(* Logix 5000 AddOnInstructionDefinition export SPEL_Above; software revision 30.01 *)

ADD_ON_INSTRUCTION SPEL_ExecCmd   (* revision 1.0 *)
// Executes a command in the robot controller.  Normally this is called by higher level AOIs.
VAR_INPUT
   Start : BOOL; {required}
   MaxTime : DINT := 3000; {required}
END_VAR
VAR_OUTPUT
   InCycle : BOOL; {access Read Only, visible}
   Done : BOOL; {access Read Only, visible}
   Error : BOOL; {access Read Only, visible}
END_VAR
VAR_IN_OUT
   ExtInputs : AB:ETHERNET_MODULE_INT_128Bytes:I:0; {required}
        .DATA[0].0   // ExtCmdGet
        .DATA[0].1   // ExtRespSet
        .DATA[0].2   // ExtCmdResult
        .DATA[0].3   // ExtError
   ExtOutputs : AB:ETHERNET_MODULE_INT_128Bytes:O:0; {required}
        .DATA[0].0   // ExtCmdSet
        .DATA[0].1   // ExtRespGet
        .DATA[0].2   // ExtCmdReset
END_VAR
VAR_INPUT
   Cmd : INT; {required}
   CmdParam1 : INT; {required}
   CmdParam2 : INT; {required}
   CmdParam3 : INT; {required}
   CmdParam4 : INT; {required}
   CmdParam5 : INT; {required}
   CmdParam6 : INT; {required}
   CmdParam7 : INT; {required}
END_VAR
VAR_OUTPUT
   CmdEcho : INT; {access Read Only, visible}
   Resp1 : INT; {access Read Only, visible}
   Resp2 : INT; {access Read Only, visible}
   Resp3 : INT; {access Read Only, visible}
   Resp4 : INT; {access Read Only, visible}
   Resp5 : INT; {access Read Only, visible}
   Resp6 : INT; {access Read Only, visible}
   Resp7 : INT; {access Read Only, visible}
   ErrCode1 : INT; {access Read Only, visible}
   ErrCode2 : INT; {access Read Only, visible}
END_VAR
VAR
   ExtReset : BOOL; {access None}
   ExtError : BOOL; {access None}
   ExtCmdSet : BOOL; {access None}   // Cmd Ready
   ExtCmdGet : BOOL; {access None}   // Cmd Received
   CmdXferDone : BOOL; {access None}
   ExtRespSet : BOOL; {access None}   // Resp Ready
   RespXferDone : BOOL; {access None}
   ExtCmdResult : BOOL; {access None}   // Normal or Error?
   TmrCmdDataRdy : TIMER := (PRE := 5); {access None}
   OneShotDoneOff : BOOL; {access None}
   OneShotStart : BOOL; {access None}
   StartInit : BOOL; {access None}
   OneShotStartError : BOOL; {access None}
   TmrCycle : TIMER := (PRE := 5000); {access None}
   OneshotTmrPreset : BOOL; {access None}
   TmrCmdSet : TIMER := (PRE := 20); {access None}
   OnShotCmdDataXfer : BOOL; {access None}
   OneShotRespDataXfer : BOOL; {access None}
   OneShotDataRdy : BOOL; {access None}
   OtherCmdInCycle : BOOL; {access None}
   s : BOOL; {access None}
   OneShotUnsetCmdIncycle : BOOL; {access None}
   OneShotSetCmdIncycle : BOOL; {access None}
   OneShotSetOtherCmdInCycleError : BOOL; {access None}
   OneShotSetBit : BOOL; {access None}
   MaxTimeError : BOOL; {access None}
END_VAR

ROUTINE Logic   (* ladder *)
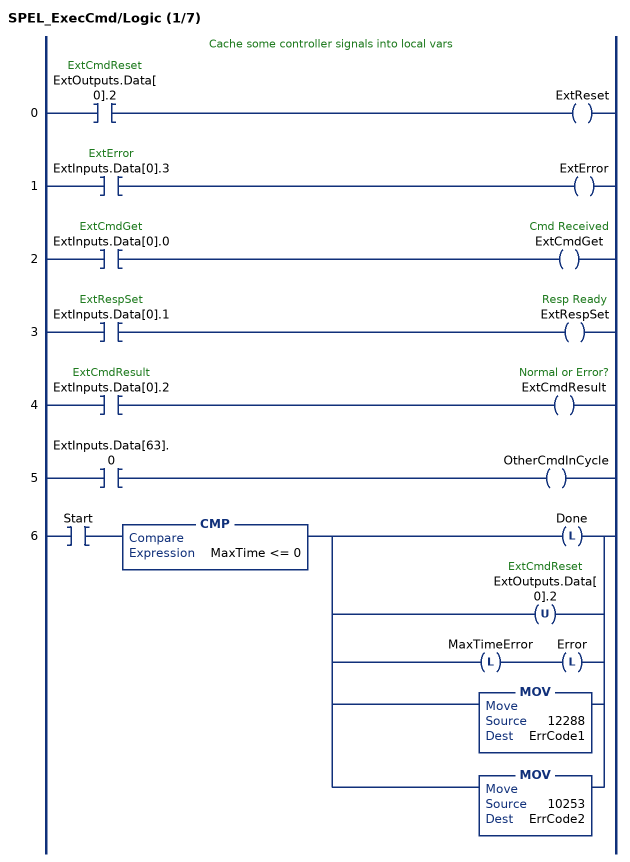
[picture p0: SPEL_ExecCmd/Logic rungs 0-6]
   // Cache some controller signals into local vars
   0: XIC(ExtOutputs.Data[0].2)OTE(ExtReset);
   1: XIC(ExtInputs.Data[0].3)OTE(ExtError);
   2: XIC(ExtInputs.Data[0].0)OTE(ExtCmdGet);
   3: XIC(ExtInputs.Data[0].1)OTE(ExtRespSet);
   4: XIC(ExtInputs.Data[0].2)OTE(ExtCmdResult);
   5: XIC(ExtInputs.Data[63].0)OTE(OtherCmdInCycle);
   6: XIC(Start)CMP(MaxTime <= 0)[OTL(Done) ,OTU(ExtOutputs.Data[0].2) ,OTL(MaxTimeError) OTL(Error) ,MOV(12288,ErrCode1) ,MOV(10253,ErrCode2) ];
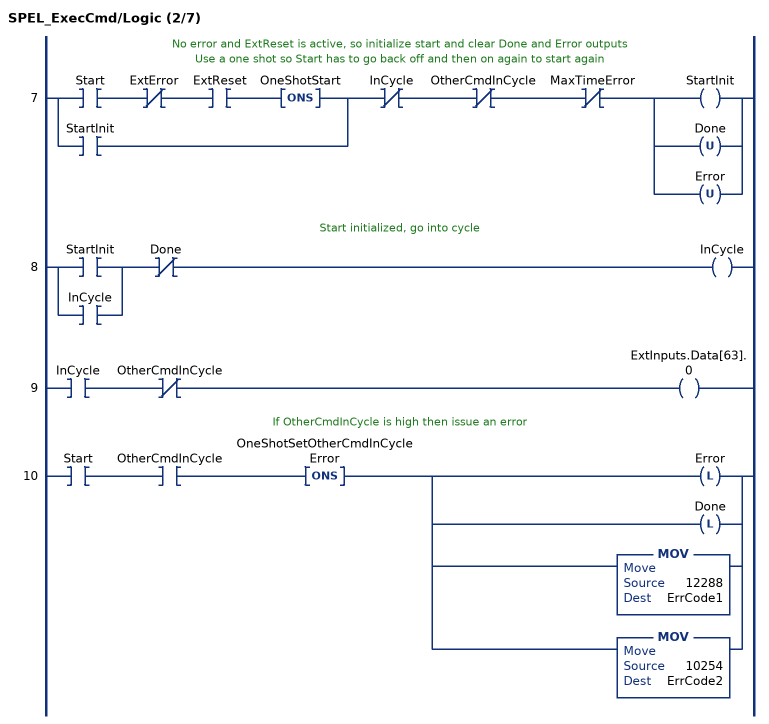
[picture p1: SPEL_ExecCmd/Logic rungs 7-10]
   // No error and ExtReset is active, so initialize start and clear Done and Error outputs
   // Use a one shot so Start has to go back off and then on again to start again
   7: [XIC(Start) XIO(ExtError) XIC(ExtReset) ONS(OneShotStart) ,XIC(StartInit) ]XIO(InCycle)XIO(OtherCmdInCycle)XIO(MaxTimeError)[OTE(StartInit) ,OTU(Done) ,OTU(Error) ];
   // Start initialized, go into cycle
   8: [XIC(StartInit) ,XIC(InCycle) ]XIO(Done)OTE(InCycle);
   9: XIC(InCycle)XIO(OtherCmdInCycle)OTE(ExtInputs.Data[63].0);
   // If OtherCmdInCycle is high then issue an error
   10: XIC(Start)XIC(OtherCmdInCycle)ONS(OneShotSetOtherCmdInCycleError)[OTL(Error) ,OTL(Done) ,MOV(12288,ErrCode1) ,MOV(10254,ErrCode2) ];
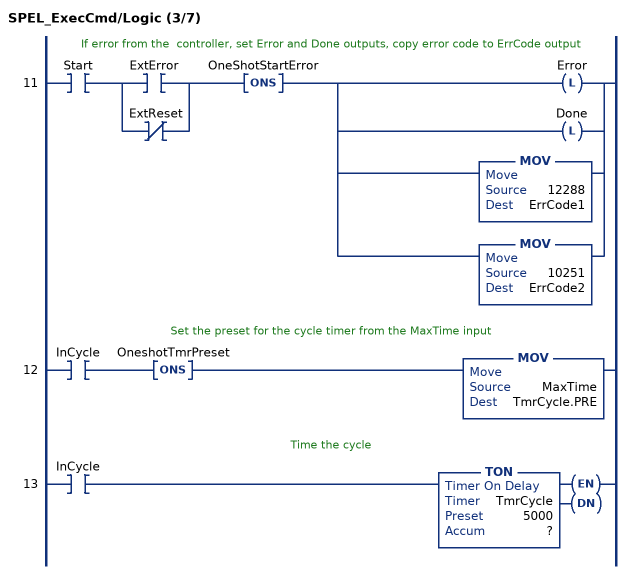
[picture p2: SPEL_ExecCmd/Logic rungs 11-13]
   // If error from the  controller, set Error and Done outputs, copy error code to ErrCode output
   11: XIC(Start)[XIC(ExtError) ,XIO(ExtReset) ]ONS(OneShotStartError)[OTL(Error) ,OTL(Done) ,MOV(12288,ErrCode1) ,MOV(10251,ErrCode2) ];
   // Set the preset for the cycle timer from the MaxTime input
   12: XIC(InCycle)ONS(OneshotTmrPreset)MOV(MaxTime,TmrCycle.PRE);
   // Time the cycle
   13: XIC(InCycle)TON(TmrCycle,?,?);
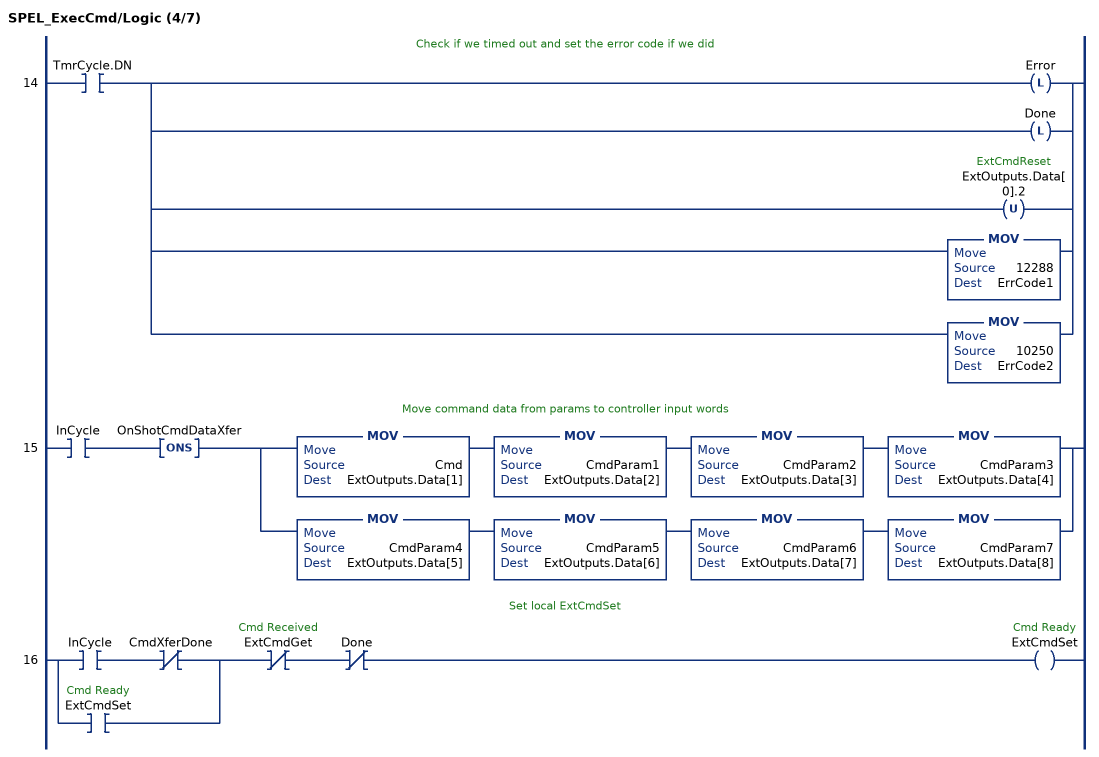
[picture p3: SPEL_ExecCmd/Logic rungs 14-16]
   // Check if we timed out and set the error code if we did
   14: XIC(TmrCycle.DN)[OTL(Error) ,OTL(Done) ,OTU(ExtOutputs.Data[0].2) ,MOV(12288,ErrCode1) ,MOV(10250,ErrCode2) ];
   // Move command data from params to controller input words
   15: XIC(InCycle)ONS(OnShotCmdDataXfer)[MOV(Cmd,ExtOutputs.Data[1]) MOV(CmdParam1,ExtOutputs.Data[2]) MOV(CmdParam2,ExtOutputs.Data[3]) MOV(CmdParam3,ExtOutputs.Data[4]) ,MOV(CmdParam4,ExtOutputs.Data[5]) MOV(CmdParam5,ExtOutputs.Data[6]) MOV(CmdParam6,ExtOutputs.Data[7]) MOV(CmdParam7,ExtOutputs.Data[8]) ];
   // Set local ExtCmdSet
   16: [XIC(InCycle) XIO(CmdXferDone) ,XIC(ExtCmdSet) ]XIO(ExtCmdGet)XIO(Done)OTE(ExtCmdSet);
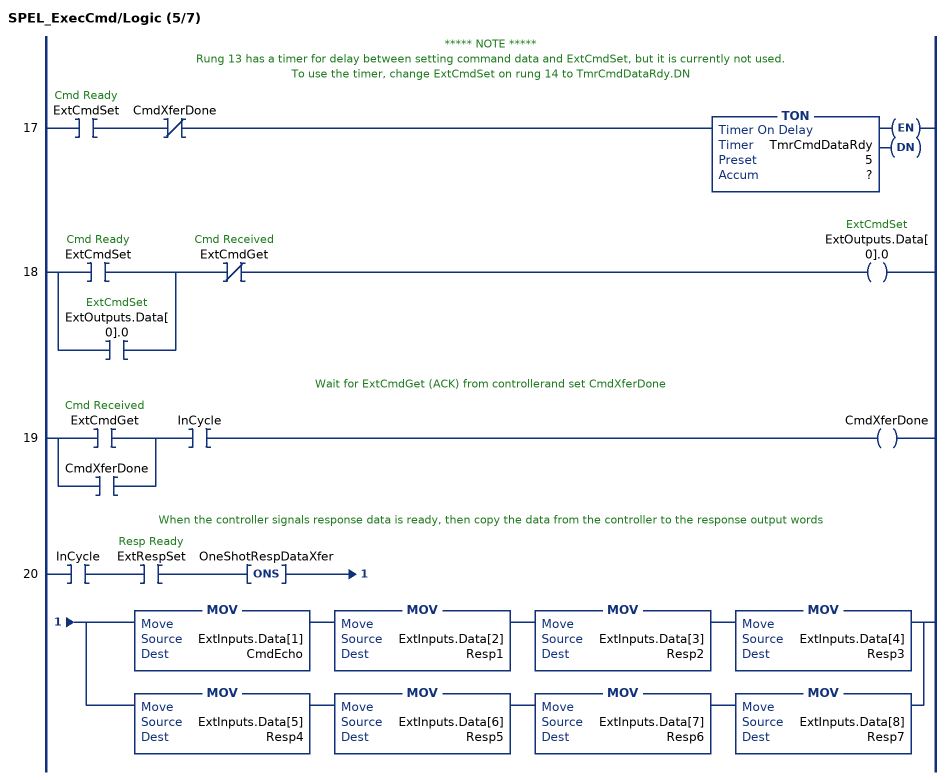
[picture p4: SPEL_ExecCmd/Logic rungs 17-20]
   // ***** NOTE *****
   // Rung 13 has a timer for delay between setting command data and ExtCmdSet, but it is currently not used.
   // To use the timer, change ExtCmdSet on rung 14 to TmrCmdDataRdy.DN
   17: XIC(ExtCmdSet)XIO(CmdXferDone)TON(TmrCmdDataRdy,?,?);
   18: [XIC(ExtCmdSet) ,XIC(ExtOutputs.Data[0].0) ]XIO(ExtCmdGet)OTE(ExtOutputs.Data[0].0);
   // Wait for ExtCmdGet (ACK) from controllerand set CmdXferDone
   19: [XIC(ExtCmdGet) ,XIC(CmdXferDone) ]XIC(InCycle)OTE(CmdXferDone);
   // When the controller signals response data is ready, then copy the data from the controller to the response output words
   20: XIC(InCycle)XIC(ExtRespSet)ONS(OneShotRespDataXfer)[MOV(ExtInputs.Data[1],CmdEcho) MOV(ExtInputs.Data[2],Resp1) MOV(ExtInputs.Data[3],Resp2) MOV(ExtInputs.Data[4],Resp3) ,MOV(ExtInputs.Data[5],Resp4) MOV(ExtInputs.Data[6],Resp5) MOV(ExtInputs.Data[7],Resp6) MOV(ExtInputs.Data[8],Resp7) ];
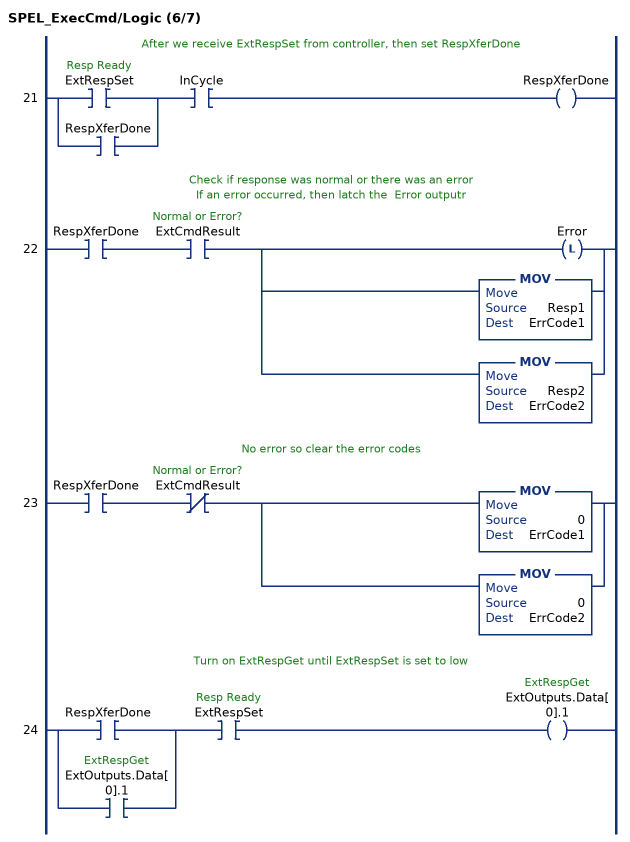
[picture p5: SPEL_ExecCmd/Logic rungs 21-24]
   // After we receive ExtRespSet from controller, then set RespXferDone
   21: [XIC(ExtRespSet) ,XIC(RespXferDone) ]XIC(InCycle)OTE(RespXferDone);
   // Check if response was normal or there was an error
   // If an error occurred, then latch the  Error outputr
   22: XIC(RespXferDone)XIC(ExtCmdResult)[OTL(Error) ,MOV(Resp1,ErrCode1) ,MOV(Resp2,ErrCode2) ];
   // No error so clear the error codes
   23: XIC(RespXferDone)XIO(ExtCmdResult)[MOV(0,ErrCode1) ,MOV(0,ErrCode2) ];
   // Turn on ExtRespGet until ExtRespSet is set to low
   24: [XIC(RespXferDone) ,XIC(ExtOutputs.Data[0].1) ]XIC(ExtRespSet)OTE(ExtOutputs.Data[0].1);
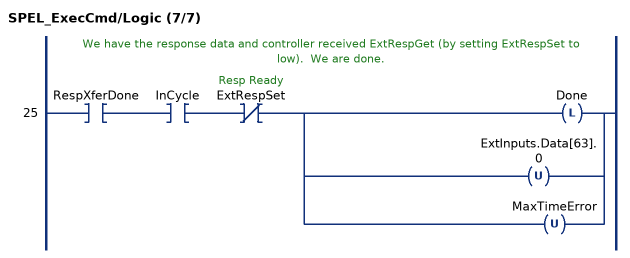
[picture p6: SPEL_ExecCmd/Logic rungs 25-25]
   // We have the response data and controller received ExtRespGet (by setting ExtRespSet to low).  We are done.
   25: XIC(RespXferDone)XIC(InCycle)XIO(ExtRespSet)[OTL(Done) ,OTU(ExtInputs.Data[63].0) ,OTU(MaxTimeError) ];
END_ROUTINE
END_ADD_ON_INSTRUCTION

ADD_ON_INSTRUCTION SPEL_Above   (* revision 1.0, vendor SEIKO EPSON CORP. *)
// Sets the elbow orientation of the specified point to ABOVE.
VAR_INPUT
   Start : BOOL; {required}
END_VAR
VAR_OUTPUT
   InCycle : BOOL; {access Read Only, visible}
   Done : BOOL; {access Read Only, visible}
   Error : BOOL; {access Read Only, visible}
END_VAR
VAR_INPUT
   Point : INT; {required}
END_VAR
VAR_IN_OUT
   ExtInputs : AB:ETHERNET_MODULE_INT_128Bytes:I:0; {required}
   ExtOutputs : AB:ETHERNET_MODULE_INT_128Bytes:O:0; {required}
END_VAR
VAR_OUTPUT
   ErrCode1 : INT; {access Read Only, visible}
   ErrCode2 : INT; {access Read Only, visible}
END_VAR
VAR
   ExecAbove : SPEL_ExecCmd := (MaxTime := 3000); {access None}
   StartCoil : BOOL; {access None}
   ExecTimeout : DINT; {access None}
   OneShotStart : BOOL; {access None}
END_VAR

ROUTINE Logic   (* ladder *)
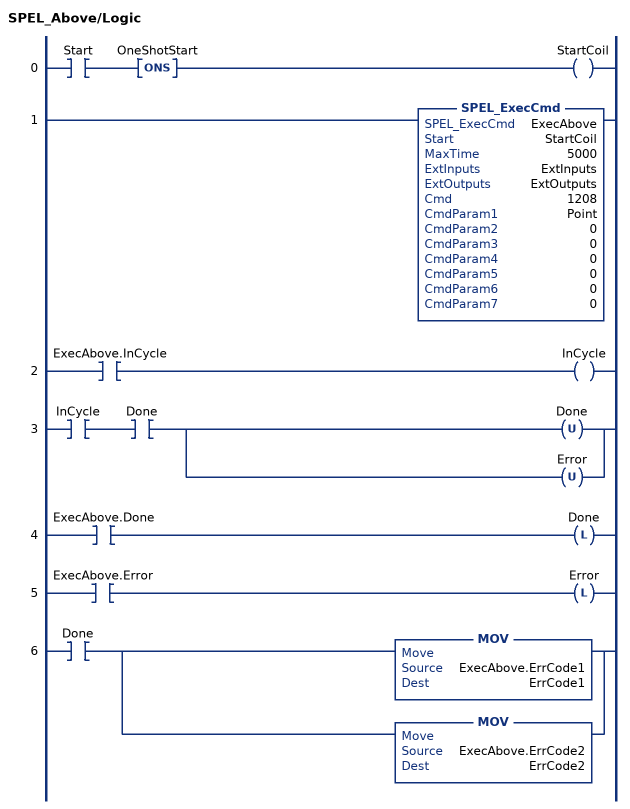
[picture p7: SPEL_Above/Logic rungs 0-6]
   0: XIC(Start)ONS(OneShotStart)OTE(StartCoil);
   1: SPEL_ExecCmd(ExecAbove,StartCoil,5000,ExtInputs,ExtOutputs,1208,Point,0,0,0,0,0,0);
   2: XIC(ExecAbove.InCycle)OTE(InCycle);
   3: XIC(InCycle)XIC(Done)[OTU(Done) ,OTU(Error) ];
   4: XIC(ExecAbove.Done)OTL(Done);
   5: XIC(ExecAbove.Error)OTL(Error);
   6: XIC(Done)[MOV(ExecAbove.ErrCode1,ErrCode1) ,MOV(ExecAbove.ErrCode2,ErrCode2) ];
END_ROUTINE
END_ADD_ON_INSTRUCTION

ADD_ON_INSTRUCTION SPEL_Accel   (* revision 1.0, vendor SEIKO EPSON CORP. *)
// Sets the point to point acceleration and deceleration for the current robot.  Accel and Decel inputs are a percentage.
VAR_INPUT
   Start : BOOL; {required}
END_VAR
VAR_OUTPUT
   InCycle : BOOL; {access Read Only, visible}
   Done : BOOL; {access Read Only, visible}
   Error : BOOL; {access Read Only, visible}
END_VAR
VAR_INPUT
   Accel : INT; {required}
   Decel : INT; {required}
END_VAR
VAR_IN_OUT
   ExtInputs : AB:ETHERNET_MODULE_INT_128Bytes:I:0; {required}
   ExtOutputs : AB:ETHERNET_MODULE_INT_128Bytes:O:0; {required}
END_VAR
VAR_OUTPUT
   ErrCode1 : INT; {access Read Only, visible}
   ErrCode2 : INT; {access Read Only, visible}
END_VAR
VAR
   ExecAccel : SPEL_ExecCmd := (MaxTime := 3000); {access None}   // Execute Accel Cmd
        .INCYCLE   // ExecInCycle
        .DONE   // ExecDone
        .ERROR   // ExecError
   OneShotStart : BOOL; {access None}
   StartCoil : BOOL; {access None}
   ExecTimeout : DINT; {access None}
END_VAR

ROUTINE Logic   (* ladder *)
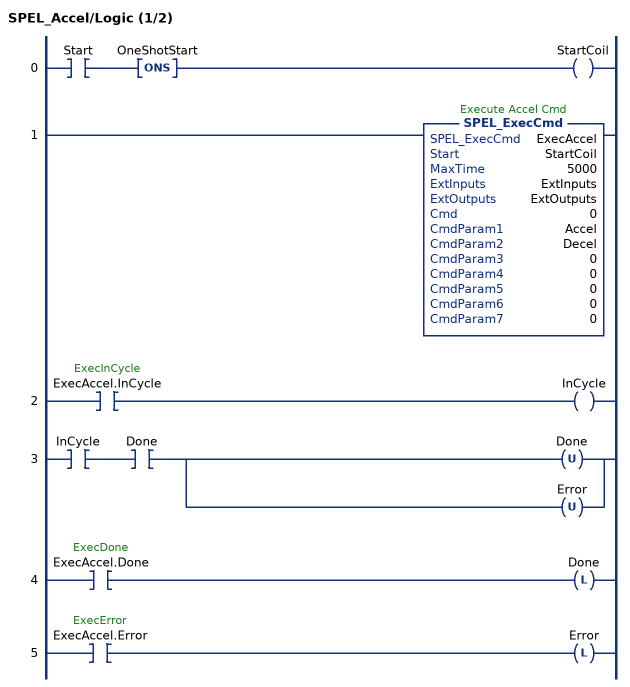
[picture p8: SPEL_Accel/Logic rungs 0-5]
   0: XIC(Start)ONS(OneShotStart)OTE(StartCoil);
   1: SPEL_ExecCmd(ExecAccel,StartCoil,5000,ExtInputs,ExtOutputs,0,Accel,Decel,0,0,0,0,0);
   2: XIC(ExecAccel.InCycle)OTE(InCycle);
   3: XIC(InCycle)XIC(Done)[OTU(Done) ,OTU(Error) ];
   4: XIC(ExecAccel.Done)OTL(Done);
   5: XIC(ExecAccel.Error)OTL(Error);
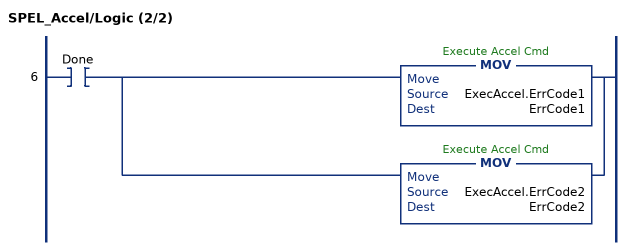
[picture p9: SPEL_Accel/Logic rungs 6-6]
   6: XIC(Done)[MOV(ExecAccel.ErrCode1,ErrCode1) ,MOV(ExecAccel.ErrCode2,ErrCode2) ];
END_ROUTINE
END_ADD_ON_INSTRUCTION

ADD_ON_INSTRUCTION SPEL_AccelS   (* revision 1.0, vendor SEIKO EPSON CORP. *)
// Sets linear motion acceleration and deceleration.
VAR_INPUT
   Start : BOOL; {required}
END_VAR
VAR_OUTPUT
   InCycle : BOOL; {access Read Only, visible}
   Done : BOOL; {access Read Only, visible}
   Error : BOOL; {access Read Only, visible}
END_VAR
VAR_INPUT
   Accel : REAL; {required}
   Decel : REAL; {required}
END_VAR
VAR_IN_OUT
   ExtInputs : AB:ETHERNET_MODULE_INT_128Bytes:I:0; {required}
   ExtOutputs : AB:ETHERNET_MODULE_INT_128Bytes:O:0; {required}
END_VAR
VAR_OUTPUT
   ErrCode1 : INT; {access Read Only, visible}
   ErrCode2 : INT; {access Read Only, visible}
END_VAR
VAR
   ExecAccelS : SPEL_ExecCmd := (MaxTime := 3000); {access None}
   Decel_INTS : INT[2]; {access None}
   Decelx1000 : DINT; {access None}
   OneShotStart : BOOL; {access None}
   StartInit : BOOL; {access None}
   Accel_INTS : INT[2]; {access None}
   Accelx1000 : DINT; {access None}
   ExecTimeout : DINT; {access None}
END_VAR

ROUTINE Logic   (* ladder *)
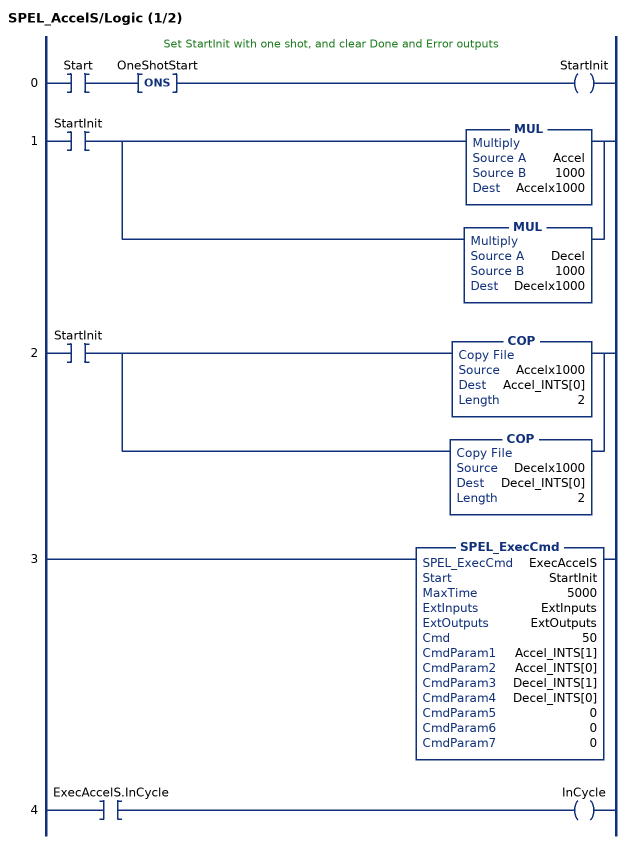
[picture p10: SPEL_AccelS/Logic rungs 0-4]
   // Set StartInit with one shot, and clear Done and Error outputs
   0: XIC(Start)ONS(OneShotStart)OTE(StartInit);
   1: XIC(StartInit)[MUL(Accel,1000,Accelx1000) ,MUL(Decel,1000,Decelx1000) ];
   2: XIC(StartInit)[COP(Accelx1000,Accel_INTS[0],2) ,COP(Decelx1000,Decel_INTS[0],2) ];
   3: SPEL_ExecCmd(ExecAccelS,StartInit,5000,ExtInputs,ExtOutputs,50,Accel_INTS[1],Accel_INTS[0],Decel_INTS[1],Decel_INTS[0],0,0,0);
   4: XIC(ExecAccelS.InCycle)OTE(InCycle);
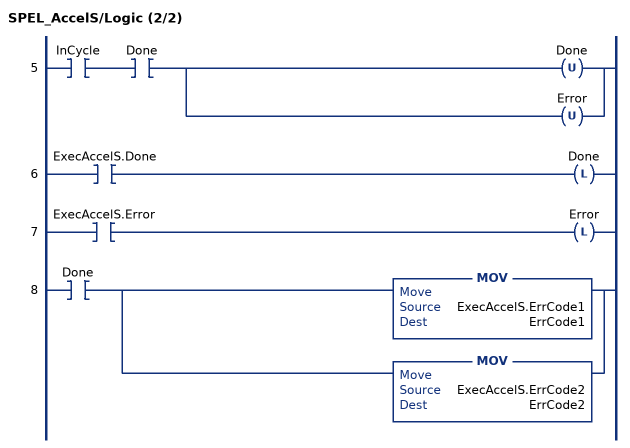
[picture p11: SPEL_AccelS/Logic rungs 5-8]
   5: XIC(InCycle)XIC(Done)[OTU(Done) ,OTU(Error) ];
   6: XIC(ExecAccelS.Done)OTL(Done);
   7: XIC(ExecAccelS.Error)OTL(Error);
   8: XIC(Done)[MOV(ExecAccelS.ErrCode1,ErrCode1) ,MOV(ExecAccelS.ErrCode2,ErrCode2) ];
END_ROUTINE
END_ADD_ON_INSTRUCTION

ADD_ON_INSTRUCTION SPEL_Arc   (* revision 1.0, vendor SEIKO EPSON CORP. *)
// Moves the arm from the current position to the specified position in circular interpolation motion on XY plane face.
VAR_INPUT
   Start : BOOL; {required}
   MaxTime : DINT := 10000; {access None, visible}
END_VAR
VAR_OUTPUT
   InCycle : BOOL; {access Read Only, visible}
   Done : BOOL; {access Read Only, visible}
   Error : BOOL; {access Read Only, visible}
END_VAR
VAR_INPUT
   MidPoint : INT; {required}
   EndPoint : INT; {required}
END_VAR
VAR_IN_OUT
   ExtInputs : AB:ETHERNET_MODULE_INT_128Bytes:I:0; {required}
   ExtOutputs : AB:ETHERNET_MODULE_INT_128Bytes:O:0; {required}
END_VAR
VAR_OUTPUT
   ErrCode1 : INT; {access Read Only, visible}
   ErrCode2 : INT; {access Read Only, visible}
END_VAR
VAR
   ExecArc : SPEL_ExecCmd := (MaxTime := 3000); {access None}
   StartCoil : BOOL; {access None}
   ExecTimeout : DINT; {access None}
   OneShotStart : BOOL; {access None}
END_VAR

ROUTINE Logic   (* ladder *)
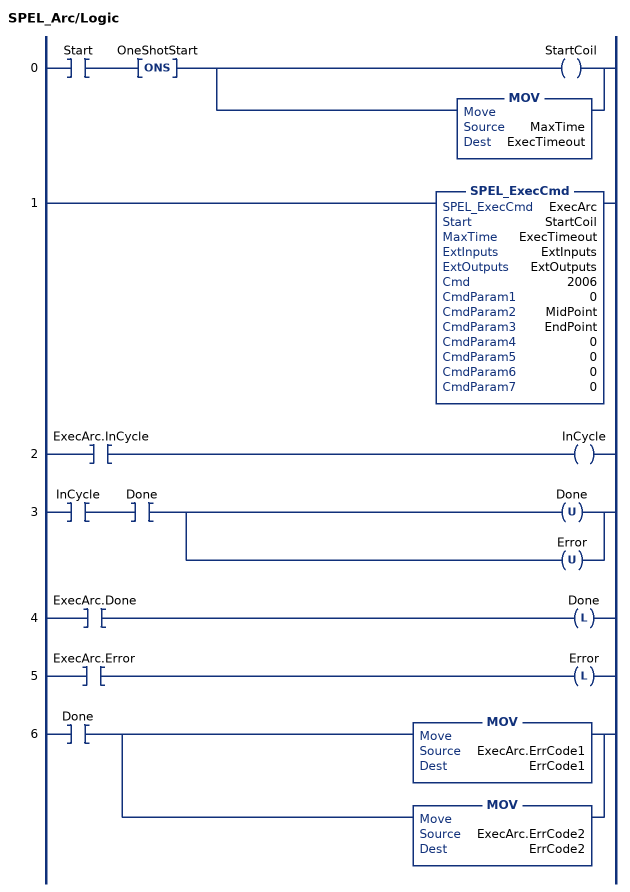
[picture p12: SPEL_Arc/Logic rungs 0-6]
   0: XIC(Start)ONS(OneShotStart)[OTE(StartCoil) ,MOV(MaxTime,ExecTimeout) ];
   1: SPEL_ExecCmd(ExecArc,StartCoil,ExecTimeout,ExtInputs,ExtOutputs,2006,0,MidPoint,EndPoint,0,0,0,0);
   2: XIC(ExecArc.InCycle)OTE(InCycle);
   3: XIC(InCycle)XIC(Done)[OTU(Done) ,OTU(Error) ];
   4: XIC(ExecArc.Done)OTL(Done);
   5: XIC(ExecArc.Error)OTL(Error);
   6: XIC(Done)[MOV(ExecArc.ErrCode1,ErrCode1) ,MOV(ExecArc.ErrCode2,ErrCode2) ];
END_ROUTINE
END_ADD_ON_INSTRUCTION

ADD_ON_INSTRUCTION SPEL_Arc3   (* revision 1.0, vendor SEIKO EPSON CORP. *)
// Moves the arm from the current position to the specified position in circular interpolation in 3 dimensions.
VAR_INPUT
   Start : BOOL; {required}
   MaxTime : DINT := 10000; {access None, visible}
END_VAR
VAR_OUTPUT
   InCycle : BOOL; {access Read Only, visible}
   Done : BOOL; {access Read Only, visible}
   Error : BOOL; {access Read Only, visible}
END_VAR
VAR_INPUT
   MidPoint : INT; {required}
   EndPoint : INT; {required}
END_VAR
VAR_IN_OUT
   ExtInputs : AB:ETHERNET_MODULE_INT_128Bytes:I:0; {required}
   ExtOutputs : AB:ETHERNET_MODULE_INT_128Bytes:O:0; {required}
END_VAR
VAR_OUTPUT
   ErrCode1 : INT; {access Read Only, visible}
   ErrCode2 : INT; {access Read Only, visible}
END_VAR
VAR
   ExecArc3 : SPEL_ExecCmd := (MaxTime := 3000); {access None}
   ExecTimeout : DINT; {access None}
   OneShotStart : BOOL; {access None}
   StartCoil : BOOL; {access None}
END_VAR

ROUTINE Logic   (* ladder *)
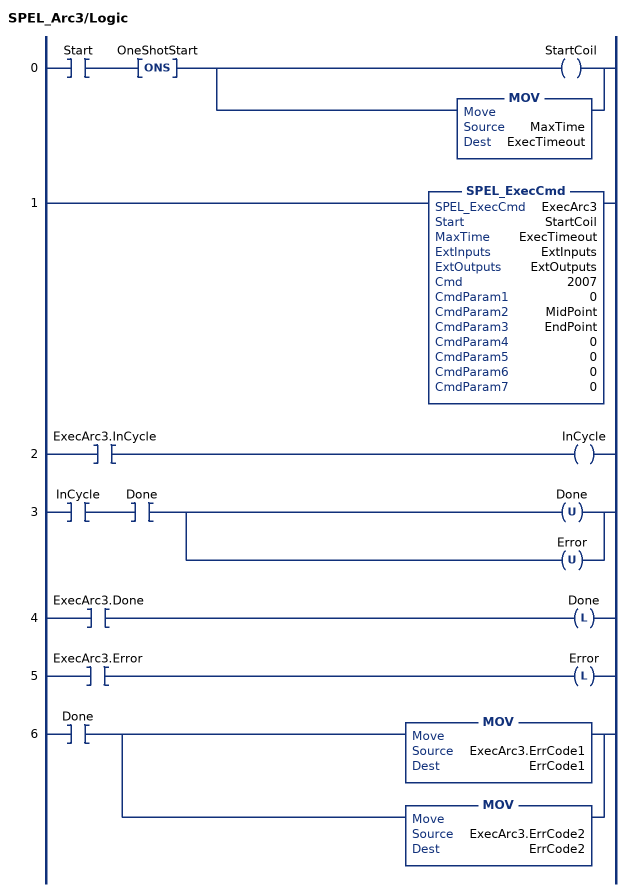
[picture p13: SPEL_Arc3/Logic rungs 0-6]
   0: XIC(Start)ONS(OneShotStart)[OTE(StartCoil) ,MOV(MaxTime,ExecTimeout) ];
   1: SPEL_ExecCmd(ExecArc3,StartCoil,ExecTimeout,ExtInputs,ExtOutputs,2007,0,MidPoint,EndPoint,0,0,0,0);
   2: XIC(ExecArc3.InCycle)OTE(InCycle);
   3: XIC(InCycle)XIC(Done)[OTU(Done) ,OTU(Error) ];
   4: XIC(ExecArc3.Done)OTL(Done);
   5: XIC(ExecArc3.Error)OTL(Error);
   6: XIC(Done)[MOV(ExecArc3.ErrCode1,ErrCode1) ,MOV(ExecArc3.ErrCode2,ErrCode2) ];
END_ROUTINE
END_ADD_ON_INSTRUCTION

ADD_ON_INSTRUCTION SPEL_ArchGet   (* revision 1.0, vendor SEIKO EPSON CORP. *)
// Gets the Arch parameter
VAR_INPUT
   Start : BOOL; {required}
END_VAR
VAR_OUTPUT
   InCycle : BOOL; {access Read Only, visible}
   Done : BOOL; {access Read Only, visible}
   Error : BOOL; {access Read Only, visible}
END_VAR
VAR_INPUT
   ArchNum : INT; {required}
END_VAR
VAR_OUTPUT
   DepartDist : REAL; {visible}
   ApproachDist : REAL; {visible}
END_VAR
VAR_IN_OUT
   ExtInputs : AB:ETHERNET_MODULE_INT_128Bytes:I:0; {required}
   ExtOutputs : AB:ETHERNET_MODULE_INT_128Bytes:O:0; {required}
END_VAR
VAR_OUTPUT
   ErrCode1 : DINT; {access Read Only, visible}
   ErrCode2 : DINT; {access Read Only, visible}
END_VAR
VAR
   Approachx1000 : DINT; {access None}
   Approach_INTS : INT[2]; {access None}
   Departx1000 : DINT; {access None}
   Depart_INTS : INT[2]; {access None}
   ExecArchGet : SPEL_ExecCmd := (MaxTime := 3000); {access None}
   OneShotStart : BOOL; {access None}
   StartCoil : BOOL; {access None}
   ExecTimeout : DINT; {access None}
END_VAR

ROUTINE Logic   (* ladder *)
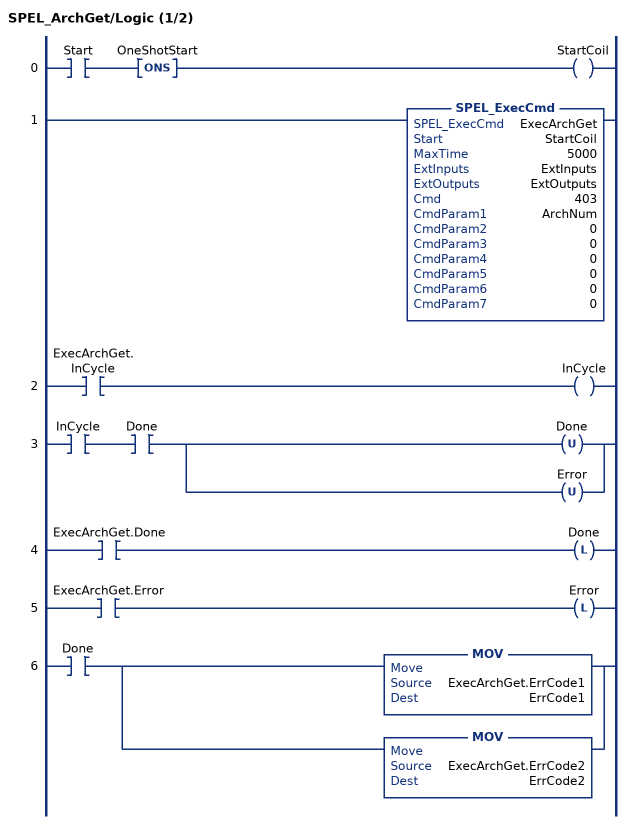
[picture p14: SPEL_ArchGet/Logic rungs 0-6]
   0: XIC(Start)ONS(OneShotStart)OTE(StartCoil);
   1: SPEL_ExecCmd(ExecArchGet,StartCoil,5000,ExtInputs,ExtOutputs,403,ArchNum,0,0,0,0,0,0);
   2: XIC(ExecArchGet.InCycle)OTE(InCycle);
   3: XIC(InCycle)XIC(Done)[OTU(Done) ,OTU(Error) ];
   4: XIC(ExecArchGet.Done)OTL(Done);
   5: XIC(ExecArchGet.Error)OTL(Error);
   6: XIC(Done)[MOV(ExecArchGet.ErrCode1,ErrCode1) ,MOV(ExecArchGet.ErrCode2,ErrCode2) ];
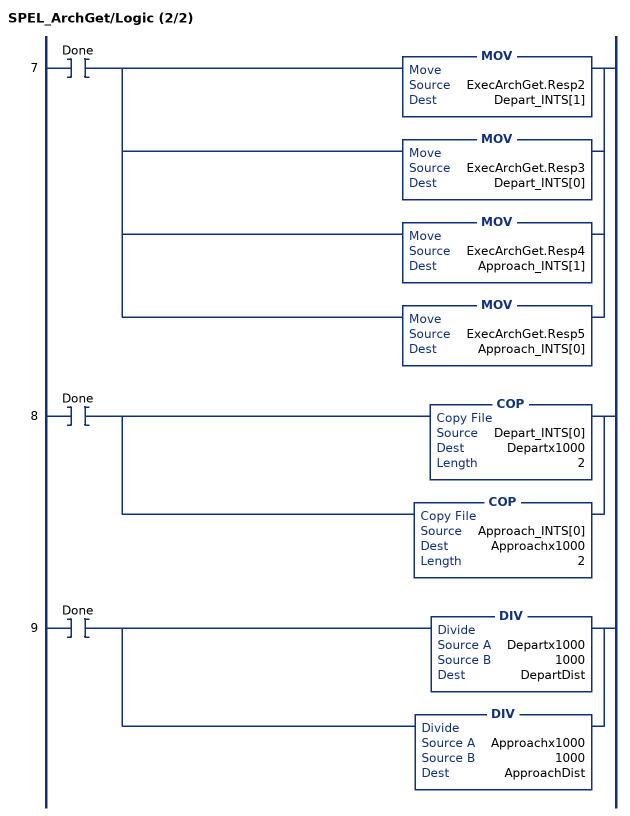
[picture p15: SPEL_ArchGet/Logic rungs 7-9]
   7: XIC(Done)[MOV(ExecArchGet.Resp2,Depart_INTS[1]) ,MOV(ExecArchGet.Resp3,Depart_INTS[0]) ,MOV(ExecArchGet.Resp4,Approach_INTS[1]) ,MOV(ExecArchGet.Resp5,Approach_INTS[0]) ];
   8: XIC(Done)[COP(Depart_INTS[0],Departx1000,2) ,COP(Approach_INTS[0],Approachx1000,2) ];
   9: XIC(Done)[DIV(Departx1000,1000,DepartDist) ,DIV(Approachx1000,1000,ApproachDist) ];
END_ROUTINE
END_ADD_ON_INSTRUCTION

ADD_ON_INSTRUCTION SPEL_ArchSet   (* revision 1.0, vendor SEIKO EPSON CORP. *)
// Sets the Arch parameter
VAR_INPUT
   Start : BOOL; {required}
END_VAR
VAR_OUTPUT
   InCycle : BOOL; {access Read Only, visible}
   Done : BOOL; {access Read Only, visible}
   Error : BOOL; {access Read Only, visible}
END_VAR
VAR_INPUT
   ArchNum : INT; {required}
   DepartDist : REAL; {visible}
   ApproachDist : REAL; {visible}
END_VAR
VAR_IN_OUT
   ExtInputs : AB:ETHERNET_MODULE_INT_128Bytes:I:0; {required}
   ExtOutputs : AB:ETHERNET_MODULE_INT_128Bytes:O:0; {required}
END_VAR
VAR_OUTPUT
   ErrCode1 : INT; {access Read Only, visible}
   ErrCode2 : INT; {access Read Only, visible}
END_VAR
VAR
   ExecArchSet : SPEL_ExecCmd := (MaxTime := 3000); {access None}
   Departx1000 : DINT; {access None}
   Depart_INTS : INT[2]; {access None}
   Approachx1000 : DINT; {access None}
   Approach_INTS : INT[2]; {access None}
   StartInit : BOOL; {access None}
   OneShotStart : BOOL; {access None}
   ExecTimeout : DINT; {access None}
END_VAR

ROUTINE Logic   (* ladder *)
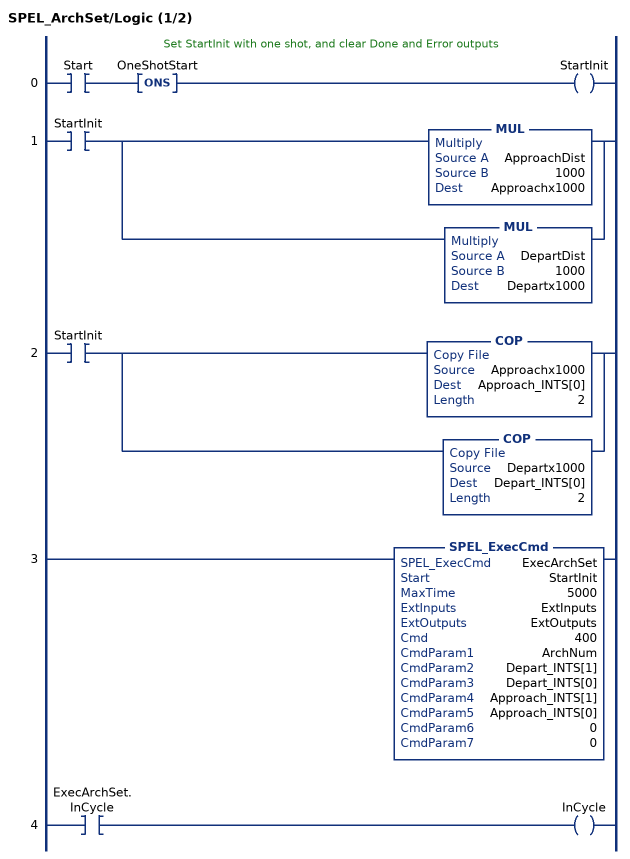
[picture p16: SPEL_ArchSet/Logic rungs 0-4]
   // Set StartInit with one shot, and clear Done and Error outputs
   0: XIC(Start)ONS(OneShotStart)OTE(StartInit);
   1: XIC(StartInit)[MUL(ApproachDist,1000,Approachx1000) ,MUL(DepartDist,1000,Departx1000) ];
   2: XIC(StartInit)[COP(Approachx1000,Approach_INTS[0],2) ,COP(Departx1000,Depart_INTS[0],2) ];
   3: SPEL_ExecCmd(ExecArchSet,StartInit,5000,ExtInputs,ExtOutputs,400,ArchNum,Depart_INTS[1],Depart_INTS[0],Approach_INTS[1],Approach_INTS[0],0,0);
   4: XIC(ExecArchSet.InCycle)OTE(InCycle);
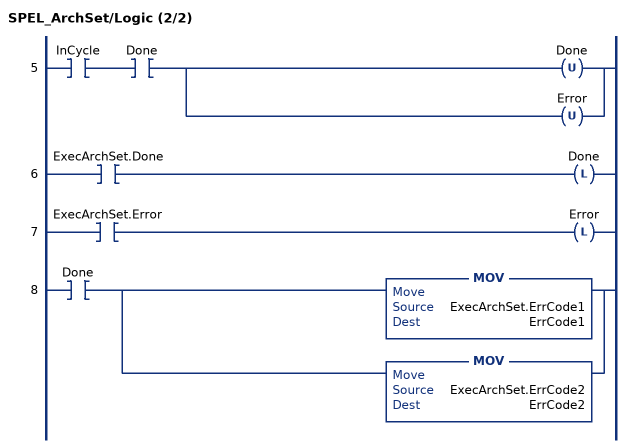
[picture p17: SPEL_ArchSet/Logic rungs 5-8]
   5: XIC(InCycle)XIC(Done)[OTU(Done) ,OTU(Error) ];
   6: XIC(ExecArchSet.Done)OTL(Done);
   7: XIC(ExecArchSet.Error)OTL(Error);
   8: XIC(Done)[MOV(ExecArchSet.ErrCode1,ErrCode1) ,MOV(ExecArchSet.ErrCode2,ErrCode2) ];
END_ROUTINE
END_ADD_ON_INSTRUCTION
